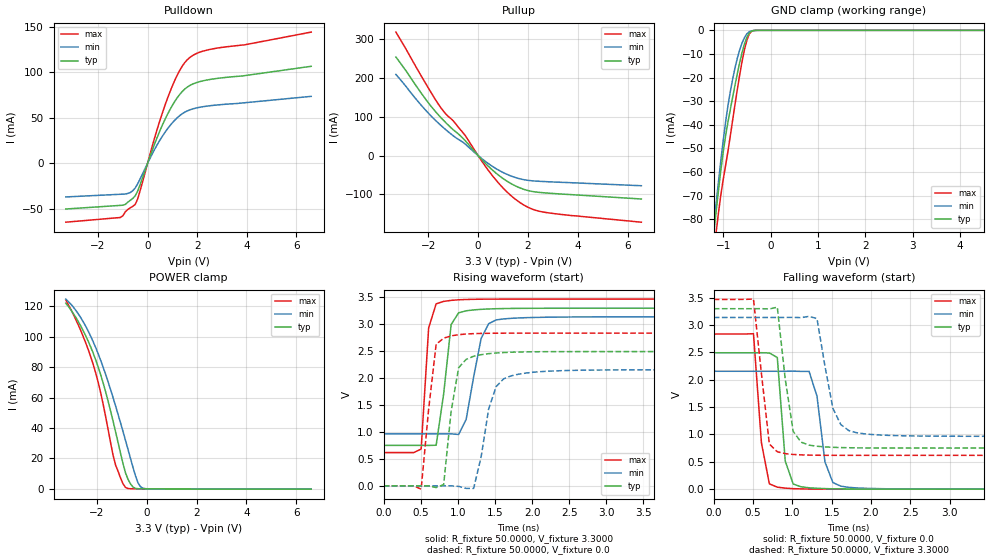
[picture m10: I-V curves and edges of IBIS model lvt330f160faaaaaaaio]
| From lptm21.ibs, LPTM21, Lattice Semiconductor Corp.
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|   Model lvt330f160faaaaaaaio
[Model]   lvt330f160faaaaaaaio
Model_type   I/O
Polarity   Non-Inverting
Enable   Active-Low
Vinl =   0.8000V
Vinh =   2.0000V
Vmeas =   1.500000V
Cref =   0.0F
Rref =   1.0000M
Vref =   0.0V
C_comp   4.2000pF   3.8000pF   7.5000pF
[Temperature Range]   25.0000   0.1050k   -40.0000
[Voltage Range]   3.3000V   3.1400V   3.4700V
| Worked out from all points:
|   slope of the pulldown table from 0 to 0.495 V, typ, clamps not added: 13.9 ohm
|   slope of the pullup table from 0 to 0.495 V, typ, clamps not added: 15.2 ohm
|   GND clamp passes 1 mA (typ) near -0.44 V on its own axis
|   POWER clamp passes 1 mA (typ) near -0.53 V on its own axis
|   rising waveform, R_fixture 50.0000, V_fixture 3.3000: 20-80 % time 132ps typ, 176ps min, 76.8ps max; typ from 0.752 V to 3.3 V
|   rising waveform, R_fixture 50.0000, V_fixture 0.0: 20-80 % time 142ps typ, 192ps min, 129ps max; typ from 0 V to 2.49 V
|   falling waveform, R_fixture 50.0000, V_fixture 0.0: 20-80 % time 82.9ps typ, 125ps min, 110ps max; typ from 2.49 V to 0 V
|   falling waveform, R_fixture 50.0000, V_fixture 3.3000: 20-80 % time 139ps typ, 180ps min, 131ps max; typ from 3.3 V to 0.752 V
[Pulldown]
|Voltage   I(typ)   I(min)   I(max)
-3.3V     -50.19mA   -36.93mA   -64.67mA
-1.1V     -46.19mA   -33.97mA   -59.5mA
-900mV    -45.15mA   -33.71mA   -53.32mA
-700mV    -40.64mA   -32.07mA   -48.88mA
-500mV    -35.7mA    -27.08mA   -45.1mA
-300mV    -23.17mA   -16.98mA   -29.79mA
300mV     22.67mA    16.24mA    29.63mA
800mV     53.75mA    37.88mA    71.35mA
1.3V      75.94mA    52.58mA    102.4mA
1.7V      85.57mA    58.78mA    116.3mA
2.5V      92.15mA    63.29mA    125.2mA
6.6V      106.7mA    73.66mA    144.3mA
[Pullup]
|Voltage   I(typ)   I(min)   I(max)
-3.3V     254.6mA    209.6mA    319mA
-2.1V     145mA      116.8mA    185.6mA
-1.5V     98.49mA    78.31mA    123.9mA
-1.3V     85.12mA    66.96mA    107.7mA
-1V       66.75mA    51.24mA    89.85mA
-600mV    44.1mA     34.07mA    58.63mA
500mV     -32.97mA   -24.66mA   -45.79mA
1V        -59.17mA   -43.58mA   -83.62mA
1.5V      -78.31mA   -56.66mA   -113mA
2.1V      -91.65mA   -64.62mA   -136.3mA
2.6V      -95.78mA   -66.79mA   -145.6mA
6.55V     -112mA     -77.75mA   -171.9mA
[GND_clamp]
|Voltage   I(typ)   I(min)   I(max)
-3.3V     -955.2mA   -930.2mA   -977.8mA
-1.2V     -86.07mA   -82.87mA   -94.72mA
-1.15V    -76.63mA   -73.23mA   -85.56mA
-1.1V     -67.6mA    -63.89mA   -77.1mA
-1V       -51.41mA   -46.51mA   -63.05mA
-900mV    -38.77mA   -31.83mA   -51.09mA
-800mV    -28.16mA   -20.53mA   -37.81mA
-700mV    -18.01mA   -11.59mA   -24.66mA
-600mV    -9.192mA   -5.229mA   -12.92mA
-450mV    -1.151mA   -576.6uA   -1.527mA
-300mV    -17.4uA    -15.66uA   -11.6uA
6.6V      0A         0A         0A
[POWER_clamp]
|Voltage   I(typ)   I(min)   I(max)
-3.25V    122.1mA    124.8mA    124.2mA
-2.65V    107.1mA    112.6mA    104.1mA
-2.35V    97.06mA    103.7mA    91.56mA
-2.05V    84.81mA    92.86mA    76.2mA
-1.65V    63.69mA    75.19mA    47.4mA
-1.35V    44.32mA    59.82mA    21.89mA
-1.25V    37.38mA    54.39mA    15.53mA
-850mV    10.3mA     31.63mA    860uA
-650mV    3.168mA    19.76mA    65.53uA
-350mV    73.34uA    3.862mA    3.121uA
-150mV    17.77uA    366.8uA    -28.16uA
6.6V      -143.8uA   -91.66uA   -226.3uA
[Ramp]
| variable   typ   min   max
dV/dt_r  1.4966/0.1403n   1.2936/0.1899n   1.7022/0.1278n
dV/dt_f  1.5290/0.1376n   1.3043/0.1782n   1.7112/0.1294n
R_load = 50.0000
[Rising Waveform]
R_fixture=   50.0000
V_fixture=   3.3000
V_fixture_min=   3.1400
V_fixture_max=   3.4700
|time   V(typ)   V(min)   V(max)
0s        751.6mV    966.1mV    618mV
505.1ps   751.7mV    966.1mV    683.2mV
606.1ps   750.6mV    966.1mV    2.934V
707.1ps   754.6mV    966.1mV    3.382V
808.1ps   1.707V     966.5mV    3.426V
909.1ps   2.998V     965.3mV    3.446V
1.111ns   3.252V     1.234V     3.462V
1.313ns   3.279V     2.738V     3.467V
1.515ns   3.291V     3.083V     3.469V
10ns      3.3V       3.14V      3.47V
[Rising Waveform]
R_fixture=   50.0000
V_fixture=   0.0
V_fixture_min=   0.0
V_fixture_max=   0.0
|time   V(typ)   V(min)   V(max)
0s        484.9nV    653.8nV    458.4nV
505.1ps   965.7nV    396.4nV    -61.92mV
707.1ps   -31.85mV   22.19uV    2.63V
808.1ps   22.23mV    16.02uV    2.743V
909.1ps   1.387V     -277.4uV   2.786V
1.01ns    2.195V     -10.24mV   2.808V
1.212ns   2.408V     -48.56mV   2.828V
1.515ns   2.468V     1.844V     2.835V
1.818ns   2.486V     2.075V     2.837V
10ns      2.494V     2.156V     2.837V
[Falling Waveform]
R_fixture=   50.0000
V_fixture=   0.0
V_fixture_min=   0.0
V_fixture_max=   0.0
|time   V(typ)   V(min)   V(max)
0s        2.494V     2.156V     2.837V
505.1ps   2.494V     2.156V     2.843V
606.1ps   2.495V     2.156V     849.6mV
808.1ps   2.408V     2.156V     36.53mV
909.1ps   515.2mV    2.156V     18.56mV
1.111ns   43.14mV    2.154V     4.92mV
1.212ns   25.35mV    2.154V     2.505mV
1.414ns   10.16mV    501mV      696.7uV
1.616ns   4.103mV    54.88mV    252.1uV
10ns      13.46uV    3.911uV    -10.62uV
[Falling Waveform]
R_fixture=   50.0000
V_fixture=   3.3000
V_fixture_min=   3.1400
V_fixture_max=   3.4700
|time   V(typ)   V(min)   V(max)
0s        3.3V       3.14V      3.47V
505.1ps   3.3V       3.14V      3.477V
707.1ps   3.295V     3.14V      824.1mV
808.1ps   3.329V     3.14V      683.9mV
909.1ps   2.014V     3.14V      649.9mV
1.01ns    1.056V     3.142V     634.8mV
1.313ns   784.9mV    3.118V     620.4mV
1.515ns   765.5mV    1.478V     618.6mV
1.818ns   755.5mV    1.032V     618.1mV
10ns      751.6mV    966.1mV    617.9mV
